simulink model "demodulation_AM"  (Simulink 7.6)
settings: Solver=ode15s  StartTime=0.0  StopTime=6e-3  RelTol=1e-3
InitFcn:
  | % amplitude et fréquence du signal modulant
  | Xm=0.2;
  | fm=1e3;
  | 
  | % amplitude et fréquence de la porteuse
  | Xp=0.5;
  | fp=50e3;
  | 
  | % taux de modulation
  | m=0.5;
  | 
  | % filtre passe bande
  | C=1e-3;
  | Q=2;
StopFcn:
  | close all, clc
  | load demodulation_AM.mat
  | plot(x(1,:),x(2,:),x(1,:),x(3,:))
  | title('Signal modulant et sortie du filtre passe bande- Modulation d''amplitude')
  | xlabel('temps')
  | grid
  | 
  | figure
  | load err_demodulation.mat
  | plot(y(1,:),y(2,:))
  | title('Erreur de démodulation')
  | xlabel('temps')
  | grid
libraries: fl_lib x31, nesl_utility x7, elec_lib x2

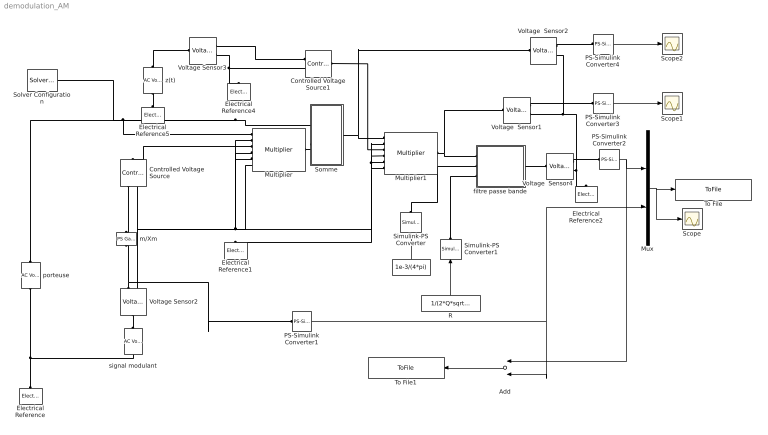
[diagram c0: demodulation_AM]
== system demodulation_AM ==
  Add : Sum  Inputs=+-
  Controlled Voltage Source : fl_lib/Electrical/Electrical Sources/Controlled Voltage Source  DialogController=NetworkEngine.DynNeDlgSource  SystemSampleTime=-1  i_Log=off  v_Log=off  LocalVarNames=|i|v  LocalVarDescs=|i|v  LocalVarLogging=[0 0]
  Controlled Voltage Source1 : fl_lib/Electrical/Electrical Sources/Controlled Voltage Source  DialogController=NetworkEngine.DynNeDlgSource  SystemSampleTime=-1  i_Log=off  v_Log=off  LocalVarNames=|i|v  LocalVarDescs=|i|v  LocalVarLogging=[0 0]
  Electrical Reference{,1..2,4..5} (5 alike) : fl_lib/Electrical/Electrical Elements/Electrical Reference  DialogController=NetworkEngine.DynNeDlgSource  SystemSampleTime=-1  i_Log=off  LocalVarNames=|i  LocalVarDescs=|i  LocalVarLogging=0
  L : Constant  Value=1e-3/(4*pi)
  Multiplier : elec_lib/Integrated Circuits/Multiplier  DialogController=NetworkEngine.DynNeDlgSource  SystemSampleTime=-1  K=1 V  A=1  Rin=1e+7 Ohm  Vdiff=15 V  Rout=0.1 Ohm  Vmin=-15 V  Vmax=15 V  Vdotmax=20 V/us  f=1 MHz  V0=0 V  LocalVarLogging=[]
  Multiplier1 : elec_lib/Integrated Circuits/Multiplier  DialogController=NetworkEngine.DynNeDlgSource  SystemSampleTime=-1  K=1 V  A=1  Rin=1e+7 Ohm  Vdiff=15 V  Rout=0.1 Ohm  Vmin=-15 V  Vmax=15 V  Vdotmax=20 V/us  f=1 MHz  V0=0 V  LocalVarLogging=[]
  Mux : Mux  Inputs=2
  PS-Simulink Converter{1..4} (4 alike) : nesl_utility/PS-Simulink Converter  DialogController=NetworkEngine.DynNeUtilDlgSource  SystemSampleTime=-1  PhysicalDomain=network_engine_domain  LeftPortType=input  RightPortType=output  SubClassName=ps_output  Unit=1  AffineConversion=off
  R : Constant  Value=1/(2*Q*sqrt(pi))
  Scope : Scope
  Scope1 : Scope
  Scope2 : Scope
  Simulink-PS Converter : nesl_utility/Simulink-PS Converter  DialogController=NetworkEngine.DynNeUtilDlgSource  SystemSampleTime=-1  PhysicalDomain=network_engine_domain  LeftPortType=input  RightPortType=output  SubClassName=ps_input  Unit=1  AffineConversion=off  InputFilterTimeConstant=.001  UdotUserProvided=0
  Simulink-PS Converter1 : nesl_utility/Simulink-PS Converter  DialogController=NetworkEngine.DynNeUtilDlgSource  SystemSampleTime=-1  PhysicalDomain=network_engine_domain  LeftPortType=input  RightPortType=output  SubClassName=ps_input  Unit=1  AffineConversion=off  InputFilterTimeConstant=.001  UdotUserProvided=0
  Solver Configuration : nesl_utility/Solver Configuration  DialogController=NetworkEngine.DynNeUtilDlgSource  SystemSampleTime=-1  PhysicalDomain=network_engine_domain  LeftPortType=input  RightPortType=generic  SubClassName=solver  Accelerate=off  Profile=off  ResidualTolerance=1e-9  MaxNonlinIter=3  MaxModeIter=2  DoFixedCost=off  UseLocalSampling=off  DoDC=off  LinearAlgebra=Sparse  LocalSolverSampleTime=.001  LocalSolverChoice=NE_BACKWARD_EULER_ADVANCER  UseLocalSolver=off
  Somme : Subsystem
  To File : ToFile  Filename=demodulation_AM.mat  MatrixName=x
  To File1 : ToFile  Filename=err_demodulation  MatrixName=y
  Voltage  Sensor1 : fl_lib/Electrical/Electrical Sensors/Voltage Sensor  DialogController=NetworkEngine.DynNeDlgSource  SystemSampleTime=-1  i1_Log=off  v1_Log=off  LocalVarNames=|i1|v1  LocalVarDescs=|i1|v1  LocalVarLogging=[0 0]
  Voltage  Sensor2 : fl_lib/Electrical/Electrical Sensors/Voltage Sensor  DialogController=NetworkEngine.DynNeDlgSource  SystemSampleTime=-1  i1_Log=off  v1_Log=off  LocalVarNames=|i1|v1  LocalVarDescs=|i1|v1  LocalVarLogging=[0 0]
  Voltage  Sensor4 : fl_lib/Electrical/Electrical Sensors/Voltage Sensor  DialogController=NetworkEngine.DynNeDlgSource  SystemSampleTime=-1  i1_Log=off  v1_Log=off  LocalVarNames=|i1|v1  LocalVarDescs=|i1|v1  LocalVarLogging=[0 0]
  Voltage Sensor2 : fl_lib/Electrical/Electrical Sensors/Voltage Sensor  DialogController=NetworkEngine.DynNeDlgSource  SystemSampleTime=-1  i1_Log=off  v1_Log=off  LocalVarNames=|i1|v1  LocalVarDescs=|i1|v1  LocalVarLogging=[0 0]
  Voltage Sensor3 : fl_lib/Electrical/Electrical Sensors/Voltage Sensor  DialogController=NetworkEngine.DynNeDlgSource  SystemSampleTime=-1  i1_Log=off  v1_Log=off  LocalVarNames=|i1|v1  LocalVarDescs=|i1|v1  LocalVarLogging=[0 0]
  filtre passe bande : Subsystem
  m/Xm : fl_lib/Physical Signals/Functions/PS Gain  DialogController=NetworkEngine.DynNeDlgSource  SystemSampleTime=-1  gain=m/Xm  LocalVarLogging=[]
  porteuse : fl_lib/Electrical/Electrical Sources/AC Voltage Source  DialogController=NetworkEngine.DynNeDlgSource  SystemSampleTime=-1  amp=Xp V  shift=0 rad  omega=fp Hz  i_Log=off  v_Log=off  LocalVarNames=|i|v  LocalVarDescs=|i|v  LocalVarLogging=[0 0]
  signal modulant : fl_lib/Electrical/Electrical Sources/AC Voltage Source  DialogController=NetworkEngine.DynNeDlgSource  SystemSampleTime=-1  amp=Xm V  shift=0 rad  omega=fm Hz  i_Log=off  v_Log=off  LocalVarNames=|i|v  LocalVarDescs=|i|v  LocalVarLogging=[0 0]
  z(t) : fl_lib/Electrical/Electrical Sources/AC Voltage Source  DialogController=NetworkEngine.DynNeDlgSource  SystemSampleTime=-1  amp=2*Xm/(m*Xp) V  shift=0 rad  omega=50 kHz  i_Log=off  v_Log=off  LocalVarNames=|i|v  LocalVarDescs=|i|v  LocalVarLogging=[0 0]
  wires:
  PS-Simulink Converter1/1 -> Mux/2, Add/2
  Mux/1 -> To File/1, Scope/1
  PS-Simulink Converter2/1 -> Mux/1, Add/1
  L/1 -> Simulink-PS Converter/1
  R/1 -> Simulink-PS Converter1/1
  PS-Simulink Converter3/1 -> Scope1/1
  PS-Simulink Converter4/1 -> Scope2/1
  Add/1 -> To File1/1
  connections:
  Multiplier/LConn1 -- Somme/LConn1 -- Solver Configuration/RConn1 -- porteuse/LConn1
  Somme/LConn2 -- Multiplier/RConn1
  porteuse/RConn1 -- Electrical Reference/LConn1 -- signal modulant/RConn1
  signal modulant/LConn1 -- Voltage Sensor2/LConn1
  Multiplier/LConn3 -- Controlled Voltage Source/LConn1
  Multiplier1/RConn1 -- filtre passe bande/LConn1 -- Voltage  Sensor1/LConn1
  Somme/RConn1 -- Multiplier1/LConn1 -- Voltage  Sensor2/LConn1
  Voltage Sensor3/RConn2 -- Electrical Reference4/LConn1 -- Controlled Voltage Source1/RConn2
  z(t)/LConn1 -- Voltage Sensor3/LConn1
  Electrical Reference5/LConn1 -- z(t)/RConn1
  filtre passe bande/RConn1 -- Voltage  Sensor4/LConn1
  Voltage  Sensor4/RConn1 -- PS-Simulink Converter2/LConn1
  Voltage  Sensor1/RConn2 -- Voltage  Sensor4/RConn2 -- Electrical Reference2/LConn1 -- Voltage  Sensor2/RConn2
  Simulink-PS Converter/RConn1 -- filtre passe bande/LConn2
  Simulink-PS Converter1/RConn1 -- filtre passe bande/LConn3
  Multiplier/LConn4 -- Multiplier/LConn2 -- Multiplier/LConn5 -- Multiplier/LConn6 -- Electrical Reference1/LConn1 -- Controlled Voltage Source/RConn2 -- Voltage Sensor2/RConn2 -- Multiplier1/LConn6 -- Multiplier1/LConn5 -- Multiplier1/LConn4 -- Multiplier1/LConn2
  Multiplier1/LConn3 -- Controlled Voltage Source1/LConn1
  Voltage  Sensor1/RConn1 -- PS-Simulink Converter3/LConn1
  Voltage  Sensor2/RConn1 -- PS-Simulink Converter4/LConn1
  Voltage Sensor3/RConn1 -- Controlled Voltage Source1/RConn1
  Controlled Voltage Source/RConn1 -- m/Xm/RConn1
  Voltage Sensor2/RConn1 -- m/Xm/LConn1 -- PS-Simulink Converter1/LConn1

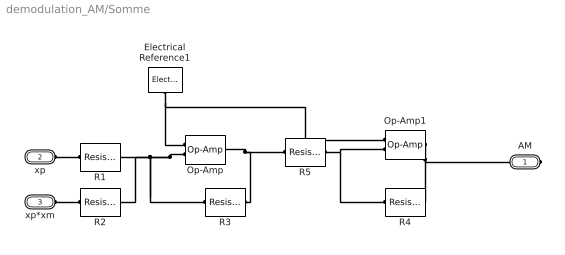
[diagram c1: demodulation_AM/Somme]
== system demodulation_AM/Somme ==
  Electrical Reference1 : fl_lib/Electrical/Electrical Elements/Electrical Reference  DialogController=NetworkEngine.DynNeDlgSource  SystemSampleTime=-1  i_Log=off  LocalVarNames=|i  LocalVarDescs=|i  LocalVarLogging=0
  Op-Amp : fl_lib/Electrical/Electrical Elements/Op-Amp  DialogController=NetworkEngine.DynNeDlgSource  SystemSampleTime=-1  i1_Log=off  v1_Log=off  outI_Log=off  LocalVarNames=|i1|v1|outI  LocalVarDescs=|i1|v1|outI  LocalVarLogging=[0 0 0]
  Op-Amp1 : fl_lib/Electrical/Electrical Elements/Op-Amp  DialogController=NetworkEngine.DynNeDlgSource  SystemSampleTime=-1  i1_Log=off  v1_Log=off  outI_Log=off  LocalVarNames=|i1|v1|outI  LocalVarDescs=|i1|v1|outI  LocalVarLogging=[0 0 0]
  R1 : fl_lib/Electrical/Electrical Elements/Resistor  DialogController=NetworkEngine.DynNeDlgSource  SystemSampleTime=-1  R=1 Ohm  i_Log=off  v_Log=off  LocalVarNames=|i|v  LocalVarDescs=|i|v  LocalVarLogging=[0 0]
  R2 : fl_lib/Electrical/Electrical Elements/Resistor  DialogController=NetworkEngine.DynNeDlgSource  SystemSampleTime=-1  R=1 Ohm  i_Log=off  v_Log=off  LocalVarNames=|i|v  LocalVarDescs=|i|v  LocalVarLogging=[0 0]
  R3 : fl_lib/Electrical/Electrical Elements/Resistor  DialogController=NetworkEngine.DynNeDlgSource  SystemSampleTime=-1  R=1 Ohm  i_Log=off  v_Log=off  LocalVarNames=|i|v  LocalVarDescs=|i|v  LocalVarLogging=[0 0]
  R4 : fl_lib/Electrical/Electrical Elements/Resistor  DialogController=NetworkEngine.DynNeDlgSource  SystemSampleTime=-1  R=1 kOhm  i_Log=off  v_Log=off  LocalVarNames=|i|v  LocalVarDescs=|i|v  LocalVarLogging=[0 0]
  R5 : fl_lib/Electrical/Electrical Elements/Resistor  DialogController=NetworkEngine.DynNeDlgSource  SystemSampleTime=-1  R=1 kOhm  i_Log=off  v_Log=off  LocalVarNames=|i|v  LocalVarDescs=|i|v  LocalVarLogging=[0 0]
  AM : PMIOPort  Port=1  Side=Right
  xp : PMIOPort  Port=2  Side=Left
  xp*xm : PMIOPort  Port=3  Side=Left
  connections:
  Electrical Reference1/LConn1 -- Op-Amp/LConn1 -- Op-Amp1/LConn1
  Op-Amp/LConn2 -- R1/RConn1 -- R2/RConn1 -- R3/LConn1
  R3/RConn1 -- Op-Amp/RConn1 -- R5/LConn1
  xp/RConn1 -- R1/LConn1
  xp*xm/RConn1 -- R2/LConn1
  Op-Amp1/RConn1 -- AM/RConn1 -- R4/RConn1
  R5/RConn1 -- Op-Amp1/LConn2 -- R4/LConn1

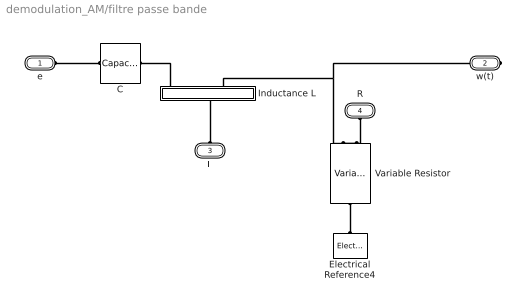
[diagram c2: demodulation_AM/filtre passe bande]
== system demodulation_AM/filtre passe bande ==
  C : fl_lib/Electrical/Electrical Elements/Capacitor  DialogController=NetworkEngine.DynNeDlgSource  SystemSampleTime=-1  c=C F  v0=0 V  r=1e-12 Ohm  g=0 1/Ohm  i_Log=off  v_Log=off  vc_Log=off  LocalVarNames=|i|v|vc  LocalVarDescs=|i|v|Internal variable for voltage across capacitor term  LocalVarLogging=[0 0 0]
  Electrical Reference4 : fl_lib/Electrical/Electrical Elements/Electrical Reference  DialogController=NetworkEngine.DynNeDlgSource  SystemSampleTime=-1  i_Log=off  LocalVarNames=|i  LocalVarDescs=|i  LocalVarLogging=0
  "Inductance L  " : Subsystem  mask{L=0}
      mask prompts: L "Inductance"
  Variable Resistor : fl_lib/Electrical/Electrical Elements/Variable Resistor  DialogController=NetworkEngine.DynNeDlgSource  SystemSampleTime=-1  Rmin=1 Ohm  i_Log=off  v_Log=off  LocalVarNames=|i|v  LocalVarDescs=|i|v  LocalVarLogging=[0 0]
  e : PMIOPort  Port=1  Side=Left
  w(t) : PMIOPort  Port=2  Side=Right
  L : PMIOPort  Port=3  Side=Left
  R : PMIOPort  Port=4  Side=Left
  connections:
  R/RConn1 -- Variable Resistor/LConn1
  L/RConn1 -- "Inductance L  "/LConn1
  "Inductance L  "/RConn2 -- w(t)/RConn1 -- Variable Resistor/LConn2
  Electrical Reference4/LConn1 -- Variable Resistor/RConn1
  C/RConn1 -- "Inductance L  "/RConn1
  e/RConn1 -- C/LConn1

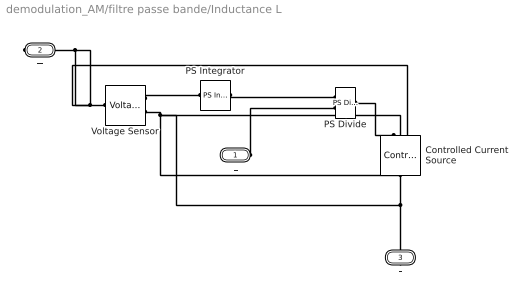
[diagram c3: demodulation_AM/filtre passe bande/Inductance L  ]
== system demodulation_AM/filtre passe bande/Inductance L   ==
  Controlled Current Source : fl_lib/Electrical/Electrical Sources/Controlled Current Source  DialogController=NetworkEngine.DynNeDlgSource  SystemSampleTime=-1  i_Log=off  v_Log=off  LocalVarNames=|i|v  LocalVarDescs=|i|v  LocalVarLogging=[0 0]
  PS Divide : fl_lib/Physical Signals/Functions/PS Divide  DialogController=NetworkEngine.DynNeDlgSource  SystemSampleTime=-1  LocalVarLogging=[]
  PS Integrator : fl_lib/Physical Signals/Linear Operators/PS Integrator  DialogController=NetworkEngine.DynNeDlgSource  SystemSampleTime=-1  x0=0  x_Log=off  LocalVarNames=|x  LocalVarDescs=|x  LocalVarLogging=0
  Voltage Sensor : fl_lib/Electrical/Electrical Sensors/Voltage Sensor  DialogController=NetworkEngine.DynNeDlgSource  SystemSampleTime=-1  i1_Log=off  v1_Log=off  LocalVarNames=|i1|v1  LocalVarDescs=|i1|v1  LocalVarLogging=[0 0]
  L : PMIOPort  Port=1  Side=Left
  + : PMIOPort  Port=2  Side=Right
  - : PMIOPort  Port=3  Side=Right
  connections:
  Voltage Sensor/RConn2 -- Controlled Current Source/LConn1 -- -/RConn1
  L/RConn1 -- PS Divide/LConn2
  Voltage Sensor/RConn1 -- PS Integrator/LConn1
  PS Integrator/RConn1 -- PS Divide/LConn1
  Voltage Sensor/LConn1 -- +/RConn1 -- Controlled Current Source/RConn2
  PS Divide/RConn1 -- Controlled Current Source/RConn1
